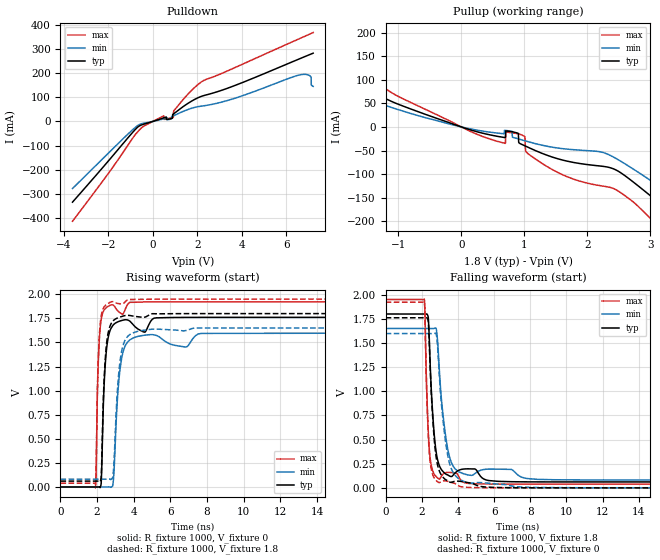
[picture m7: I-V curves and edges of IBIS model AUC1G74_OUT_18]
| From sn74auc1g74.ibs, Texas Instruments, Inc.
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[Model]   AUC1G74_OUT_18
Model_type  Output
Vref =   0
Rref =   1000
Cref =   30p
Vmeas =   0.9
| variable   typ   min   max
C_comp   5.92pF   0.26pF   17.58pF
| C_pullup   5.52pF   0.26pF   17.58pF
| C_pulldown   6.33pF   3.48pF   15.98pF
[Temperature Range]   40   100   -40
| Ambient temperature   25   85   -40
[Voltage range]   1.8   1.65   1.95
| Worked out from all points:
|   slope of the pulldown table from 0 to 0.27 V, typ, clamps not added: 34.2 ohm
|   slope of the pullup table from 0 to 0.27 V, typ, clamps not added: 24.5 ohm
|   rising waveform, R_fixture 1000, V_fixture 0: 20-80 % time 229ps typ, 331ps min, 157ps max; typ from 0 V to 1.76 V
|   falling waveform, R_fixture 1000, V_fixture 1.8: 20-80 % time 337ps typ, 509ps min, 206ps max; typ from 1.8 V to 0.061 V
|   rising waveform, R_fixture 1000, V_fixture 1.8: 20-80 % time 225ps typ, 320ps min, 155ps max; typ from 0.061 V to 1.8 V
|   falling waveform, R_fixture 1000, V_fixture 0: 20-80 % time 338ps typ, 519ps min, 205ps max; typ from 1.76 V to 0 V
[Pulldown]
| AUC1G74_OUT_18
|   Voltage   I(typ)   I(min)   I(max)
-3.6V     -334.1mA   -277.8mA   -413.4mA
-460mV    -12.94mA   -8.507mA   -23.02mA
495mV     15.07mA    10.85mA    23.55mA
855mV     12.62mA    20.1mA     15.47mA
925mV     30.87mA    22.97mA    17.67mA
955mV     32.82mA    24.27mA    45.35mA
2.265V    106.4mA    64.55mA    168.5mA
6.595V    259.7mA    192.8mA    343.3mA
7.055V    277.3mA    188.9mA    362.2mA
7.11V     279.4mA    180.2mA    364.4mA
7.115V    279.6mA    151mA      364.6mA
7.2V      282.8mA    145.3mA    368.1mA
[Pullup]
| AUC1G74_OUT_18
|   Voltage   I(typ)   I(min)   I(max)
-3.6V     269.8mA    228.7mA    318.8mA
-3.03V    214.4mA    176.4mA    261.7mA
-2.52V    166.6mA    133.1mA    210.5mA
-1.045V   50.54mA    38.59mA    67.88mA
460mV     -16.98mA   -11.23mA   -25.96mA
960mV     -37.06mA   -27.45mA   -17.13mA
1.025V    -41.05mA   -29.97mA   -52.45mA
1.28V     -55.97mA   -38.75mA   -77.3mA
2.41V     -88.67mA   -63.62mA   -130.4mA
3.155V    -162.8mA   -127.1mA   -214.7mA
3.995V    -254.8mA   -204.1mA   -324.7mA
7.2V      -602.1mA   -502.3mA   -732.1mA
[Ramp]
| AUC1G74_OUT_18
| variable   typ   min   max
dV/dt_r   1.06/2.30E-10   0.96/3.36E-10   1.16/1.57E-10
dV/dt_f   1.04/3.41E-10   0.94/5.11E-10   1.15/2.08E-10
R_load = 1000
[Rising Waveform]
| AUC1G74_OUT_18
R_fixture =   1000
C_fixture =   0
L_fixture =   0
V_fixture =   0
V_fixture_min = 0
V_fixture_max = 0
|   Time   V(typ)   V(min)   V(max)
0s        8.892nV    30.7nV     1.165nV
1.905ns   -7.573uV   -31.61nV   -9.082mV
2.15ns    -4.479mV   -3.678uV   1.609V
2.23ns    66.61mV    -6.809uV   1.745V
2.435ns   1.239V     -8.784uV   1.85V
2.675ns   1.605V     804.8uV    1.883V
2.89ns    1.684V     73.63mV    1.886V
3.305ns   1.726V     1.296V     1.802V
3.95ns    1.689V     1.545V     1.917V
20ns      1.761V     1.597V     1.922V
[Falling Waveform]
| AUC1G74_OUT_18
R_fixture =   1000
C_fixture =   0
L_fixture =   0
V_fixture =   1.8
V_fixture_min = 1.65
V_fixture_max = 1.95
|   Time   V(typ)   V(min)   V(max)
0s        1.8V       1.65V      1.95V
2.14ns    1.8V       1.65V      1.954V
2.28ns    1.801V     1.65V      964.5mV
2.42ns    1.509V     1.65V      388.1mV
2.655ns   627mV      1.65V      152.3mV
2.81ns    352.3mV    1.634V     113.9mV
2.94ns    245.8mV    1.317V     93.96mV
3.455ns   131.3mV    383.1mV    160.2mV
4.205ns   191.8mV    153.5mV    69.72mV
20ns      61.1mV     81.12mV    38.7mV
[Rising Waveform]
| AUC1G74_OUT_18
R_fixture =   1000
C_fixture =   0
L_fixture =   0
V_fixture =   1.8
V_fixture_min = 1.65
V_fixture_max = 1.95
|   Time   V(typ)   V(min)   V(max)
0s        61.05mV    81.09mV    38.68mV
1.905ns   61.04mV    81.09mV    29.67mV
2.04ns    61.25mV    81.09mV    1.182V
2.155ns   55.8mV     81.09mV    1.66V
2.44ns    1.312V     81.09mV    1.882V
2.71ns    1.672V     80.23mV    1.917V
2.89ns    1.727V     167.3mV    1.923V
3.285ns   1.766V     1.349V     1.899V
3.91ns    1.776V     1.596V     1.946V
20ns      1.8V       1.65V      1.95V
[Falling Waveform]
| AUC1G74_OUT_18
R_fixture =   1000
C_fixture =   0
L_fixture =   0
V_fixture =   0
V_fixture_min = 0
V_fixture_max = 0
|   Time   V(typ)   V(min)   V(max)
0s        1.761V     1.597V     1.922V
2.14ns    1.761V     1.597V     1.926V
2.28ns    1.762V     1.597V     941.1mV
2.42ns    1.467V     1.597V     349.7mV
2.655ns   579.3mV    1.598V     112.2mV
2.92ns    201.9mV    1.32V      56.52mV
3.13ns    120.2mV    778.9mV    71.5mV
3.47ns    67.86mV    303mV      65.53mV
4.35ns    61.16mV    64.72mV    7.307mV
20ns      51.82uV    23.23uV    22.42uV
